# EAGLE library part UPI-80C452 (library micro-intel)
MICROCOMPUTER/PERIPHERAL DEVICE
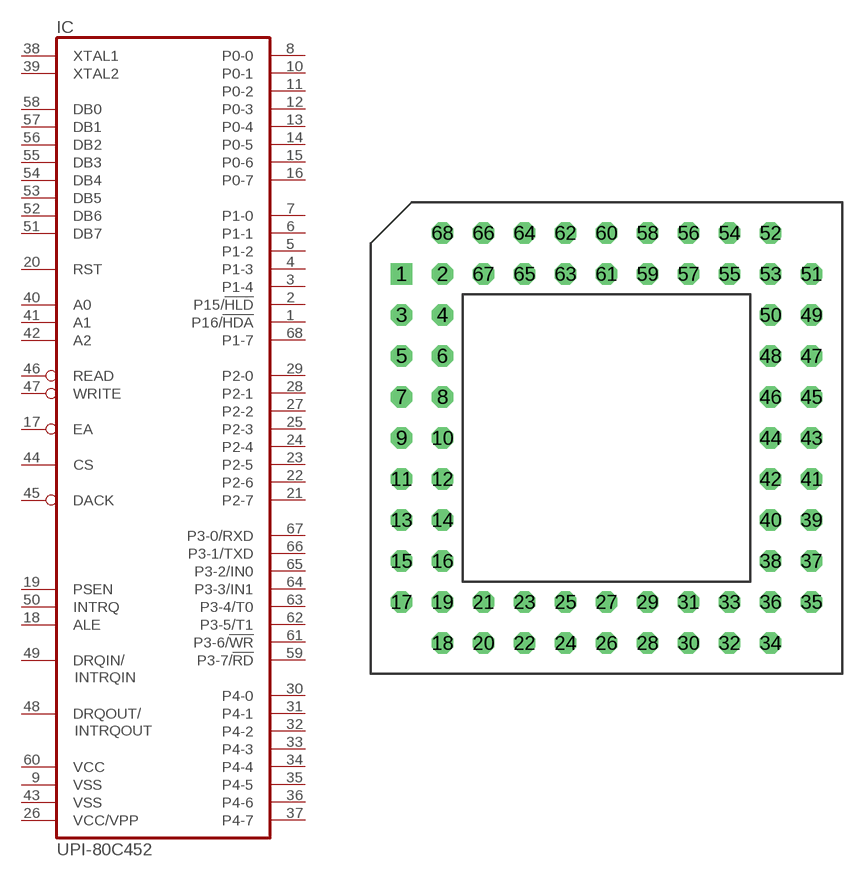
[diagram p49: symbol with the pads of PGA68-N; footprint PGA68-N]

Designator prefix IC

## UPI-80C452 (OC_FARNELL: unknown; OC_NEWARK: unknown)  [PGA68-N]
1  P16/!HDA
2  P15/!HLD
3  P1-4
4  P1-3
5  P1-2
6  P1-1
7  P1-0
8  P0-0
9  VSS  pwr
10  P0-1
11  P0-2
12  P0-3
13  P0-4
14  P0-5
15  P0-6
16  P0-7
17  EA  in
18  ALE  out
19  PSEN  out
20  RST  in
21  P2-7
22  P2-6
23  P2-5
24  P2-4
25  P2-3
26  VCC/VPP  pwr
27  P2-2
28  P2-1
29  P2-0
30  P4-0
31  P4-1
32  P4-2
33  P4-3
34  P4-4
35  P4-5
36  P4-6
37  P4-7
38  XTAL1  in
39  XTAL2  out
40  A0  in
41  A1  in
42  A2  in
43  VSS  pwr
44  CS  in
45  DACK  in
46  READ  in
47  WRITE  in
48  DRQOUT/  out
49  DRQIN/  out
50  INTRQ  out
51  DB7
52  DB6
53  DB5
54  DB4
55  DB3
56  DB2
57  DB1
58  DB0
59  P3-7/!RD
60  VCC  pwr
61  P3-6/!WR
62  P3-5/T1
63  P3-4/T0
64  P3-3/IN1
65  P3-2/IN0
66  P3-1/TXD
67  P3-0/RXD
68  P1-7

## Footprint PGA68-N (pad centres in mm)
Pin Grid Array
drill 0.813 square: 1 -12.7,10.16
drill 0.813 octagon: 2 -10.16,10.16; 3 -12.7,7.62; 4 -10.16,7.62; 5 -12.7,5.08; 6 -10.16,5.08; 7 -12.7,2.54; 8 -10.16,2.54; 9 -12.7,0; 10 -10.16,0; 11 -12.7,-2.54; 12 -10.16,-2.54; 13 -12.7,-5.08; 14 -10.16,-5.08; 15 -12.7,-7.62; 16 -10.16,-7.62; 17 -12.7,-10.16; 18 -10.16,-12.7; 19 -10.16,-10.16; 20 -7.62,-12.7; 21 -7.62,-10.16; 22 -5.08,-12.7; 23 -5.08,-10.16; 24 -2.54,-12.7; 25 -2.54,-10.16; 26 0,-12.7; 27 0,-10.16; 28 2.54,-12.7; 29 2.54,-10.16; 30 5.08,-12.7; 31 5.08,-10.16; 32 7.62,-12.7; 33 7.62,-10.16; 34 10.16,-12.7; 35 12.7,-10.16; 36 10.16,-10.16; 37 12.7,-7.62; 38 10.16,-7.62; 39 12.7,-5.08; 40 10.16,-5.08; 41 12.7,-2.54; 42 10.16,-2.54; 43 12.7,0; 44 10.16,0; 45 12.7,2.54; 46 10.16,2.54; 47 12.7,5.08; 48 10.16,5.08; 49 12.7,7.62; 50 10.16,7.62; 51 12.7,10.16; 52 10.16,12.7; 53 10.16,10.16; 54 7.62,12.7; 55 7.62,10.16; 56 5.08,12.7; 57 5.08,10.16; 58 2.54,12.7; 59 2.54,10.16; 60 0,12.7; 61 0,10.16; 62 -2.54,12.7; 63 -2.54,10.16; 64 -5.08,12.7; 65 -5.08,10.16; 66 -7.62,12.7; 67 -7.62,10.16; 68 -10.16,12.7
